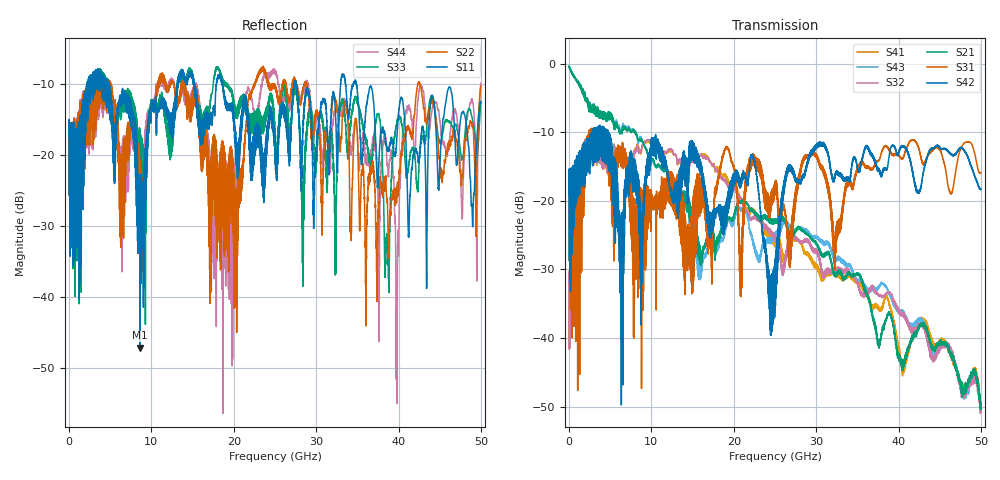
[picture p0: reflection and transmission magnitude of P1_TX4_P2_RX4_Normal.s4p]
!Keysight Technologies,N5225A,MY51441389,A.10.49.11
!Date: Monday, July 08, 2019 11:22:02
!Correction: S11(Full 4 Port(1,2,3,4))
!S12(Full 4 Port(1,2,3,4))
!S13(Full 4 Port(1,2,3,4))
!S14(Full 4 Port(1,2,3,4))
!S21(Full 4 Port(1,2,3,4))
!S22(Full 4 Port(1,2,3,4))
!S23(Full 4 Port(1,2,3,4))
!S24(Full 4 Port(1,2,3,4))
!S31(Full 4 Port(1,2,3,4))
!S32(Full 4 Port(1,2,3,4))
!S33(Full 4 Port(1,2,3,4))
!S34(Full 4 Port(1,2,3,4))
!S41(Full 4 Port(1,2,3,4))
!S42(Full 4 Port(1,2,3,4))
!S43(Full 4 Port(1,2,3,4))
!S44(Full 4 Port(1,2,3,4))
!S4P File: Measurements: <S11,S12,S13,S14>,
!<S21,S22,S23,S24>,
!<S31,S32,S33,S34>,
!<S41,S42,S43,S44>:
# Hz S  dB  R 50
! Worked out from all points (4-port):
!   5000 points, 10 MHz to 50 GHz, reference 50 ohm
!   strongest paths, dB at 10 MHz, 12.51 GHz, 25.01 GHz, 37.51 GHz, 50 GHz:
!     S42: -19.0, -18.8, -36.2, -15.5, -18.3
!     S31: -19.1, -15.9, -18.1, -14.3, -15.9
!     S21: -0.4, -17.3, -23.0, -40.7, -49.9
!     S32: -32.8, -12.7, -25.9, -33.5, -50.3
!     S43: -0.4, -17.4, -24.9, -32.6, -50.6
!     S41: -33.0, -12.9, -26.6, -35.4, -50.3
!   lowest |S11| = -47.2 dB at 8.64 GHz (marker M1), VSWR 1.01, Z = 49.6 - j0.19 ohm
!   |S11| at or under -10 dB: 4.824 GHz to 13.13 GHz (8.306 GHz wide, 92.5 % of centre); 18.65 GHz to 27.32 GHz (8.673 GHz wide, 37.7 % of centre); 34.89 GHz to end of sweep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
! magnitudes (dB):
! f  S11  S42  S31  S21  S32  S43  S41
! 10 MHz  -17.4  -19.0  -19.1  -0.4  -32.8  -0.4  -33.0
! 8.64 GHz  -47.2  -23.0  -21.6  -11.3  -12.8  -11.0  -12.7
! 24.94 GHz  -17.8  -29.5  -17.8  -23.1  -25.0  -25.3  -25.9
! 38.6 GHz  -19.3  -15.3  -12.2  -37.0  -33.4  -32.7  -33.9
! 39.8 GHz  -17.4  -13.1  -13.1  -41.9  -35.5  -36.0  -40.4
! 41.05 GHz  -23.6  -12.9  -12.2  -41.9  -37.5  -37.4  -42.3
! 50 GHz  -12.6  -18.3  -15.9  -49.9  -50.3  -50.6  -50.3
